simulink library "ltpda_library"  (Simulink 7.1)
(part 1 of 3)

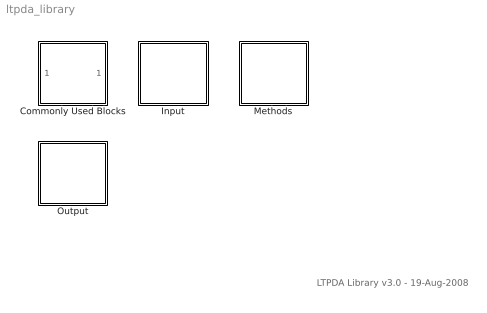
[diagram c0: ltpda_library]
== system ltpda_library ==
  note: LTPDA Library v3.0 - 19-Aug-2008
  Commonly Used Blocks : Subsystem
  Input : Subsystem
  Methods : Subsystem  Tag=subsystem  AncestorBlock=libraryBase/SubSystName
  Output : Subsystem

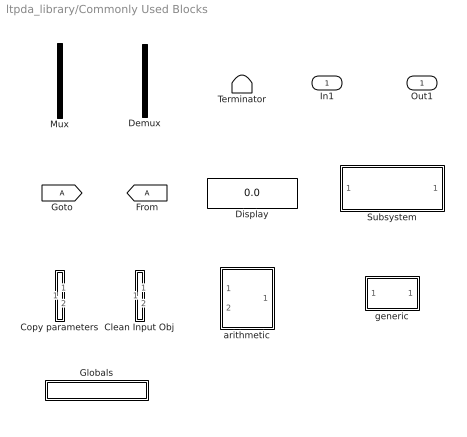
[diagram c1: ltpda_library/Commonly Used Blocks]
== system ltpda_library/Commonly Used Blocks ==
  In1 : Inport  OutDataType=sfix(16)  OutScaling=2^0
  Clean Input Obj : Subsystem
  Copy parameters : Subsystem
  Demux : Demux  Tag=demux  Outputs=2
  Display : Display
  Globals : Subsystem  Tag=globals
  Mux : Mux  Tag=mux  Inputs=2
  Subsystem : Subsystem
  Terminator : Terminator
  arithmetic : Subsystem  Tag=arithmetic
  generic : Subsystem  Tag=function
  Out1 : Outport  OutDataType=sfix(16)  OutScaling=2^0

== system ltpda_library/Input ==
  Object from list : Subsystem  Tag=input

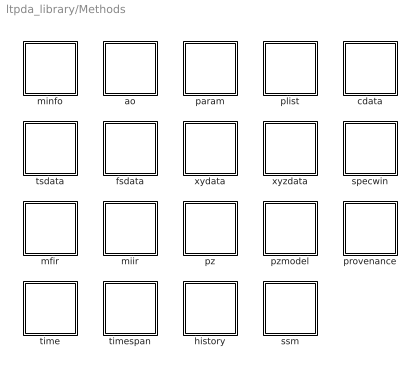
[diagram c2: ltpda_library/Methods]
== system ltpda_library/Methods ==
  ao : Subsystem  Tag=subsystem  AncestorBlock=libraryBase/SubSystName
  cdata : Subsystem  Tag=subsystem  AncestorBlock=libraryBase/SubSystName
  fsdata : Subsystem  Tag=subsystem  AncestorBlock=libraryBase/SubSystName
  history : Subsystem  Tag=subsystem  AncestorBlock=libraryBase/SubSystName
  mfir : Subsystem  Tag=subsystem  AncestorBlock=libraryBase/SubSystName
  miir : Subsystem  Tag=subsystem  AncestorBlock=libraryBase/SubSystName
  minfo : Subsystem  Tag=subsystem  AncestorBlock=libraryBase/SubSystName
  param : Subsystem  Tag=subsystem  AncestorBlock=libraryBase/SubSystName
  plist : Subsystem  Tag=subsystem  AncestorBlock=libraryBase/SubSystName
  provenance : Subsystem  Tag=subsystem  AncestorBlock=libraryBase/SubSystName
  pz : Subsystem  Tag=subsystem  AncestorBlock=libraryBase/SubSystName
  pzmodel : Subsystem  Tag=subsystem  AncestorBlock=libraryBase/SubSystName
  specwin : Subsystem  Tag=subsystem  AncestorBlock=libraryBase/SubSystName
  ssm : Subsystem  Tag=subsystem  AncestorBlock=libraryBase/SubSystName
  time : Subsystem  Tag=subsystem  AncestorBlock=libraryBase/SubSystName
  timespan : Subsystem  Tag=subsystem  AncestorBlock=libraryBase/SubSystName
  tsdata : Subsystem  Tag=subsystem  AncestorBlock=libraryBase/SubSystName
  xydata : Subsystem  Tag=subsystem  AncestorBlock=libraryBase/SubSystName
  xyzdata : Subsystem  Tag=subsystem  AncestorBlock=libraryBase/SubSystName

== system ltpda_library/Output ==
  Send to output : Subsystem
  iplot : Subsystem  Tag=method ao
  plot : Subsystem  Tag=method ao
  save : Subsystem  Tag=method ao

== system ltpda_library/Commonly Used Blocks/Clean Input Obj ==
  In1 : Inport  OutDataType=sfix(16)  OutScaling=2^0
  In2 : Inport  Port=2  OutDataType=sfix(16)  OutScaling=2^0
  cleaninput : M-S-Function  FunctionName=g_cleaninput
  Out1 : Outport  OutDataType=sfix(16)  OutScaling=2^0
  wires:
  In2/1 -> cleaninput/2
  In1/1 -> cleaninput/1
  cleaninput/1 -> Out1/1

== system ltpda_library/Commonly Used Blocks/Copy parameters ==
  In1 : Inport  OutDataType=sfix(16)  OutScaling=2^0
  In2 : Inport  Port=2  OutDataType=sfix(16)  OutScaling=2^0
  copyparam : M-S-Function  FunctionName=g_copyparams
  Out1 : Outport  OutDataType=sfix(16)  OutScaling=2^0
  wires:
  copyparam/1 -> Out1/1
  In1/1 -> copyparam/1
  In2/1 -> copyparam/2

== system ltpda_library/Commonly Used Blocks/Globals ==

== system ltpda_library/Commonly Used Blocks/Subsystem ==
  In1 : Inport  OutDataType=sfix(16)  OutScaling=2^0
  Out1 : Outport  OutDataType=sfix(16)  OutScaling=2^0

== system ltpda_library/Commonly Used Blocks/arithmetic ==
  alpha : Inport  Tag=1  OutDataType=sfix(16)  OutScaling=2^0
  beta : Inport  Tag=2  Port=2  OutDataType=sfix(16)  OutScaling=2^0
  Mux : Mux  Tag=mux  Inputs=2
  arithmetic_func : M-S-Function  Tag=arithmetic  FunctionName=ltpdasim
  Out1 : Outport  OutDataType=sfix(16)  OutScaling=2^0
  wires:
  arithmetic_func/1 -> Out1/1
  Mux/1 -> arithmetic_func/1
  alpha/1 -> Mux/1
  beta/1 -> Mux/2

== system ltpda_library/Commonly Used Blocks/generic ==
  In1 : Inport  OutDataType=sfix(16)  OutScaling=2^0
  generic : M-S-Function  Tag=generic  FunctionName=ltpdasim
  Out1 : Outport  OutDataType=sfix(16)  OutScaling=2^0
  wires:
  generic/1 -> Out1/1
  In1/1 -> generic/1

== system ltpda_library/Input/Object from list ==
  Input : Constant  Value=0  OutDataType=sfix(16)  OutScaling=2^0
  Input AO : Outport  OutDataType=sfix(16)  OutScaling=2^0
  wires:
  Input/1 -> Input AO/1

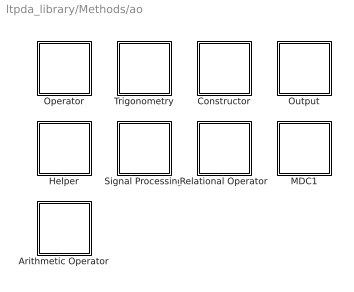
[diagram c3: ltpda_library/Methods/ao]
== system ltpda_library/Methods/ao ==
  Arithmetic Operator : Subsystem  Tag=subsystem  AncestorBlock=libraryBase/SubSystName
  Constructor : Subsystem  Tag=subsystem  AncestorBlock=libraryBase/SubSystName
  Helper : Subsystem  Tag=subsystem  AncestorBlock=libraryBase/SubSystName
  MDC1 : Subsystem  Tag=subsystem  AncestorBlock=libraryBase/SubSystName
  Operator : Subsystem  Tag=subsystem  AncestorBlock=libraryBase/SubSystName
  Output : Subsystem  Tag=subsystem  AncestorBlock=libraryBase/SubSystName
  Relational Operator : Subsystem  Tag=subsystem  AncestorBlock=libraryBase/SubSystName
  Signal Processing : Subsystem  Tag=subsystem  AncestorBlock=libraryBase/SubSystName
  Trigonometry : Subsystem  Tag=subsystem  AncestorBlock=libraryBase/SubSystName

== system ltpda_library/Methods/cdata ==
  Constructor : Subsystem  Tag=subsystem  AncestorBlock=libraryBase/SubSystName
  Helper : Subsystem  Tag=subsystem  AncestorBlock=libraryBase/SubSystName
  Output : Subsystem  Tag=subsystem  AncestorBlock=libraryBase/SubSystName
  Relational Operator : Subsystem  Tag=subsystem  AncestorBlock=libraryBase/SubSystName

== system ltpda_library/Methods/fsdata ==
  Constructor : Subsystem  Tag=subsystem  AncestorBlock=libraryBase/SubSystName
  Helper : Subsystem  Tag=subsystem  AncestorBlock=libraryBase/SubSystName
  Output : Subsystem  Tag=subsystem  AncestorBlock=libraryBase/SubSystName
  Relational Operator : Subsystem  Tag=subsystem  AncestorBlock=libraryBase/SubSystName

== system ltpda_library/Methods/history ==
  Constructor : Subsystem  Tag=subsystem  AncestorBlock=libraryBase/SubSystName
  Helper : Subsystem  Tag=subsystem  AncestorBlock=libraryBase/SubSystName
  Output : Subsystem  Tag=subsystem  AncestorBlock=libraryBase/SubSystName
  Relational Operator : Subsystem  Tag=subsystem  AncestorBlock=libraryBase/SubSystName

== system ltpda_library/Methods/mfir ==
  Constructor : Subsystem  Tag=subsystem  AncestorBlock=libraryBase/SubSystName
  Helper : Subsystem  Tag=subsystem  AncestorBlock=libraryBase/SubSystName
  Output : Subsystem  Tag=subsystem  AncestorBlock=libraryBase/SubSystName
  Relational Operator : Subsystem  Tag=subsystem  AncestorBlock=libraryBase/SubSystName
  Signal Processing : Subsystem  Tag=subsystem  AncestorBlock=libraryBase/SubSystName

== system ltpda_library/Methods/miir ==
  Constructor : Subsystem  Tag=subsystem  AncestorBlock=libraryBase/SubSystName
  Helper : Subsystem  Tag=subsystem  AncestorBlock=libraryBase/SubSystName
  Output : Subsystem  Tag=subsystem  AncestorBlock=libraryBase/SubSystName
  Relational Operator : Subsystem  Tag=subsystem  AncestorBlock=libraryBase/SubSystName
  Signal Processing : Subsystem  Tag=subsystem  AncestorBlock=libraryBase/SubSystName

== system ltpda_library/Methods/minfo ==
  Constructor : Subsystem  Tag=subsystem  AncestorBlock=libraryBase/SubSystName
  Helper : Subsystem  Tag=subsystem  AncestorBlock=libraryBase/SubSystName
  Output : Subsystem  Tag=subsystem  AncestorBlock=libraryBase/SubSystName
  Relational Operator : Subsystem  Tag=subsystem  AncestorBlock=libraryBase/SubSystName

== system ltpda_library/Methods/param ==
  Constructor : Subsystem  Tag=subsystem  AncestorBlock=libraryBase/SubSystName
  Helper : Subsystem  Tag=subsystem  AncestorBlock=libraryBase/SubSystName
  Output : Subsystem  Tag=subsystem  AncestorBlock=libraryBase/SubSystName
  Relational Operator : Subsystem  Tag=subsystem  AncestorBlock=libraryBase/SubSystName

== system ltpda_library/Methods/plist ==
  Constructor : Subsystem  Tag=subsystem  AncestorBlock=libraryBase/SubSystName
  Helper : Subsystem  Tag=subsystem  AncestorBlock=libraryBase/SubSystName
  Output : Subsystem  Tag=subsystem  AncestorBlock=libraryBase/SubSystName
  Relational Operator : Subsystem  Tag=subsystem  AncestorBlock=libraryBase/SubSystName
  Signal Processing : Subsystem  Tag=subsystem  AncestorBlock=libraryBase/SubSystName

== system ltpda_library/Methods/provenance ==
  Constructor : Subsystem  Tag=subsystem  AncestorBlock=libraryBase/SubSystName
  Helper : Subsystem  Tag=subsystem  AncestorBlock=libraryBase/SubSystName
  Output : Subsystem  Tag=subsystem  AncestorBlock=libraryBase/SubSystName
  Relational Operator : Subsystem  Tag=subsystem  AncestorBlock=libraryBase/SubSystName

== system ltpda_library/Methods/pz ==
  Constructor : Subsystem  Tag=subsystem  AncestorBlock=libraryBase/SubSystName
  Helper : Subsystem  Tag=subsystem  AncestorBlock=libraryBase/SubSystName
  Output : Subsystem  Tag=subsystem  AncestorBlock=libraryBase/SubSystName
  Relational Operator : Subsystem  Tag=subsystem  AncestorBlock=libraryBase/SubSystName
  Signal Processing : Subsystem  Tag=subsystem  AncestorBlock=libraryBase/SubSystName

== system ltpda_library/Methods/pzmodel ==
  Constructor : Subsystem  Tag=subsystem  AncestorBlock=libraryBase/SubSystName
  Helper : Subsystem  Tag=subsystem  AncestorBlock=libraryBase/SubSystName
  Operator : Subsystem  Tag=subsystem  AncestorBlock=libraryBase/SubSystName
  Output : Subsystem  Tag=subsystem  AncestorBlock=libraryBase/SubSystName
  Relational Operator : Subsystem  Tag=subsystem  AncestorBlock=libraryBase/SubSystName
  Signal Processing : Subsystem  Tag=subsystem  AncestorBlock=libraryBase/SubSystName

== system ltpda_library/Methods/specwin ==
  Constructor : Subsystem  Tag=subsystem  AncestorBlock=libraryBase/SubSystName
  Helper : Subsystem  Tag=subsystem  AncestorBlock=libraryBase/SubSystName
  Output : Subsystem  Tag=subsystem  AncestorBlock=libraryBase/SubSystName
  Relational Operator : Subsystem  Tag=subsystem  AncestorBlock=libraryBase/SubSystName

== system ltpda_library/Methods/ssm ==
  Constructor : Subsystem  Tag=subsystem  AncestorBlock=libraryBase/SubSystName
  Helper : Subsystem  Tag=subsystem  AncestorBlock=libraryBase/SubSystName
  Output : Subsystem  Tag=subsystem  AncestorBlock=libraryBase/SubSystName
  Relational Operator : Subsystem  Tag=subsystem  AncestorBlock=libraryBase/SubSystName
  STATESPACE : Subsystem  Tag=subsystem  AncestorBlock=libraryBase/SubSystName

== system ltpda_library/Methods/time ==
  Arithmetic Operator : Subsystem  Tag=subsystem  AncestorBlock=libraryBase/SubSystName
  Constructor : Subsystem  Tag=subsystem  AncestorBlock=libraryBase/SubSystName
  Helper : Subsystem  Tag=subsystem  AncestorBlock=libraryBase/SubSystName
  Output : Subsystem  Tag=subsystem  AncestorBlock=libraryBase/SubSystName
  Relational Operator : Subsystem  Tag=subsystem  AncestorBlock=libraryBase/SubSystName

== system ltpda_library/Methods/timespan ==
  Constructor : Subsystem  Tag=subsystem  AncestorBlock=libraryBase/SubSystName
  Helper : Subsystem  Tag=subsystem  AncestorBlock=libraryBase/SubSystName
  Output : Subsystem  Tag=subsystem  AncestorBlock=libraryBase/SubSystName
  Relational Operator : Subsystem  Tag=subsystem  AncestorBlock=libraryBase/SubSystName

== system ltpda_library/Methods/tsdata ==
  Constructor : Subsystem  Tag=subsystem  AncestorBlock=libraryBase/SubSystName
  Helper : Subsystem  Tag=subsystem  AncestorBlock=libraryBase/SubSystName
  Output : Subsystem  Tag=subsystem  AncestorBlock=libraryBase/SubSystName
  Relational Operator : Subsystem  Tag=subsystem  AncestorBlock=libraryBase/SubSystName

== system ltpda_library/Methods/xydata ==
  Constructor : Subsystem  Tag=subsystem  AncestorBlock=libraryBase/SubSystName
  Helper : Subsystem  Tag=subsystem  AncestorBlock=libraryBase/SubSystName
  Output : Subsystem  Tag=subsystem  AncestorBlock=libraryBase/SubSystName
  Relational Operator : Subsystem  Tag=subsystem  AncestorBlock=libraryBase/SubSystName

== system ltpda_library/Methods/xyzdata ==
  Constructor : Subsystem  Tag=subsystem  AncestorBlock=libraryBase/SubSystName
  Helper : Subsystem  Tag=subsystem  AncestorBlock=libraryBase/SubSystName
  Output : Subsystem  Tag=subsystem  AncestorBlock=libraryBase/SubSystName
  Relational Operator : Subsystem  Tag=subsystem  AncestorBlock=libraryBase/SubSystName

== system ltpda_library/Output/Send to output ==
  In1 : Inport  OutDataType=sfix(16)  OutScaling=2^0
  save result : M-S-Function  FunctionName=g_saveresult
  Out1 : Outport  OutDataType=sfix(16)  OutScaling=2^0
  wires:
  In1/1 -> save result/1
  save result/1 -> Out1/1

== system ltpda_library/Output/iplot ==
  In1 : Inport  OutDataType=sfix(16)  OutScaling=2^0
  Terminator : Terminator
  iplot : M-S-Function  Tag=iplot  FunctionName=ltpdasim
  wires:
  In1/1 -> iplot/1
  iplot/1 -> Terminator/1

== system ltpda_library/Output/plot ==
  In1 : Inport  OutDataType=sfix(16)  OutScaling=2^0
  Terminator : Terminator
  plot : M-S-Function  Tag=plot  FunctionName=ltpdasim
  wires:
  In1/1 -> plot/1
  plot/1 -> Terminator/1

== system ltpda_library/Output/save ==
  In1 : Inport  OutDataType=sfix(16)  OutScaling=2^0
  Terminator : Terminator
  save : M-S-Function  Tag=save  FunctionName=ltpdasim
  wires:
  In1/1 -> save/1
  save/1 -> Terminator/1

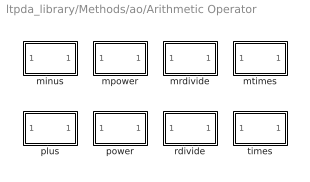
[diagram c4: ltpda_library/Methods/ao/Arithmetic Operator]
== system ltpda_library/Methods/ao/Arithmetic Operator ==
  minus : Subsystem  Tag=method ao  AncestorBlock=libraryBase/function
  mpower : Subsystem  Tag=method ao  AncestorBlock=libraryBase/function
  mrdivide : Subsystem  Tag=method ao  AncestorBlock=libraryBase/function
  mtimes : Subsystem  Tag=method ao  AncestorBlock=libraryBase/function
  plus : Subsystem  Tag=method ao  AncestorBlock=libraryBase/function
  power : Subsystem  Tag=method ao  AncestorBlock=libraryBase/function
  rdivide : Subsystem  Tag=method ao  AncestorBlock=libraryBase/function
  times : Subsystem  Tag=method ao  AncestorBlock=libraryBase/function

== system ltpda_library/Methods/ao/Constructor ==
  ao : Subsystem  Tag=method ao  AncestorBlock=libraryBase/constructor

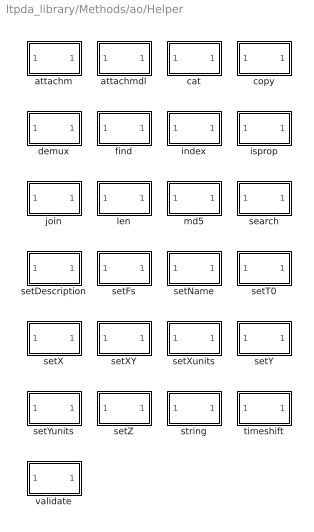
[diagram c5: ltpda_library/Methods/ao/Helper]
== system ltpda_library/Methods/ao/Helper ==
  attachm : Subsystem  Tag=method ao  AncestorBlock=libraryBase/function
  attachmdl : Subsystem  Tag=method ao  AncestorBlock=libraryBase/function
  cat : Subsystem  Tag=method ao  AncestorBlock=libraryBase/function
  copy : Subsystem  Tag=method ao  AncestorBlock=libraryBase/function
  demux : Subsystem  Tag=method ao  AncestorBlock=libraryBase/function
  find : Subsystem  Tag=method ao  AncestorBlock=libraryBase/function
  index : Subsystem  Tag=method ao  AncestorBlock=libraryBase/function
  isprop : Subsystem  Tag=method ao  AncestorBlock=libraryBase/function
  join : Subsystem  Tag=method ao  AncestorBlock=libraryBase/function
  len : Subsystem  Tag=method ao  AncestorBlock=libraryBase/function
  md5 : Subsystem  Tag=method ao  AncestorBlock=libraryBase/function
  search : Subsystem  Tag=method ao  AncestorBlock=libraryBase/function
  setDescription : Subsystem  Tag=method ao  AncestorBlock=libraryBase/function
  setFs : Subsystem  Tag=method ao  AncestorBlock=libraryBase/function
  setName : Subsystem  Tag=method ao  AncestorBlock=libraryBase/function
  setT0 : Subsystem  Tag=method ao  AncestorBlock=libraryBase/function
  setX : Subsystem  Tag=method ao  AncestorBlock=libraryBase/function
  setXY : Subsystem  Tag=method ao  AncestorBlock=libraryBase/function
  setXunits : Subsystem  Tag=method ao  AncestorBlock=libraryBase/function
  setY : Subsystem  Tag=method ao  AncestorBlock=libraryBase/function
  setYunits : Subsystem  Tag=method ao  AncestorBlock=libraryBase/function
  setZ : Subsystem  Tag=method ao  AncestorBlock=libraryBase/function
  string : Subsystem  Tag=method ao  AncestorBlock=libraryBase/function
  timeshift : Subsystem  Tag=method ao  AncestorBlock=libraryBase/function
  validate : Subsystem  Tag=method ao  AncestorBlock=libraryBase/function

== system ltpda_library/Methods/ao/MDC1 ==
  mdc1_ifo2acc_fd : Subsystem  Tag=method ao  AncestorBlock=libraryBase/function
  mdc1_ifo2acc_inloop : Subsystem  Tag=method ao  AncestorBlock=libraryBase/function
  mdc1_ifo2control : Subsystem  Tag=method ao  AncestorBlock=libraryBase/function
  mdc1_x2acc : Subsystem  Tag=method ao  AncestorBlock=libraryBase/function

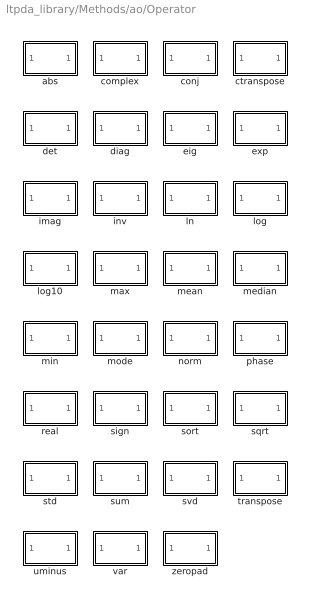
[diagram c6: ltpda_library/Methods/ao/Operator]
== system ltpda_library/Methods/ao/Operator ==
  abs : Subsystem  Tag=method ao  AncestorBlock=libraryBase/function
  complex : Subsystem  Tag=method ao  AncestorBlock=libraryBase/function
  conj : Subsystem  Tag=method ao  AncestorBlock=libraryBase/function
  ctranspose : Subsystem  Tag=method ao  AncestorBlock=libraryBase/function
  det : Subsystem  Tag=method ao  AncestorBlock=libraryBase/function
  diag : Subsystem  Tag=method ao  AncestorBlock=libraryBase/function
  eig : Subsystem  Tag=method ao  AncestorBlock=libraryBase/function
  exp : Subsystem  Tag=method ao  AncestorBlock=libraryBase/function
  imag : Subsystem  Tag=method ao  AncestorBlock=libraryBase/function
  inv : Subsystem  Tag=method ao  AncestorBlock=libraryBase/function
  ln : Subsystem  Tag=method ao  AncestorBlock=libraryBase/function
  log : Subsystem  Tag=method ao  AncestorBlock=libraryBase/function
  log10 : Subsystem  Tag=method ao  AncestorBlock=libraryBase/function
  max : Subsystem  Tag=method ao  AncestorBlock=libraryBase/function
  mean : Subsystem  Tag=method ao  AncestorBlock=libraryBase/function
  median : Subsystem  Tag=method ao  AncestorBlock=libraryBase/function
  min : Subsystem  Tag=method ao  AncestorBlock=libraryBase/function
  mode : Subsystem  Tag=method ao  AncestorBlock=libraryBase/function
  norm : Subsystem  Tag=method ao  AncestorBlock=libraryBase/function
  phase : Subsystem  Tag=method ao  AncestorBlock=libraryBase/function
  real : Subsystem  Tag=method ao  AncestorBlock=libraryBase/function
  sign : Subsystem  Tag=method ao  AncestorBlock=libraryBase/function
  sort : Subsystem  Tag=method ao  AncestorBlock=libraryBase/function
  sqrt : Subsystem  Tag=method ao  AncestorBlock=libraryBase/function
  std : Subsystem  Tag=method ao  AncestorBlock=libraryBase/function
  sum : Subsystem  Tag=method ao  AncestorBlock=libraryBase/function
  svd : Subsystem  Tag=method ao  AncestorBlock=libraryBase/function
  transpose : Subsystem  Tag=method ao  AncestorBlock=libraryBase/function
  uminus : Subsystem  Tag=method ao  AncestorBlock=libraryBase/function
  var : Subsystem  Tag=method ao  AncestorBlock=libraryBase/function
  zeropad : Subsystem  Tag=method ao  AncestorBlock=libraryBase/function

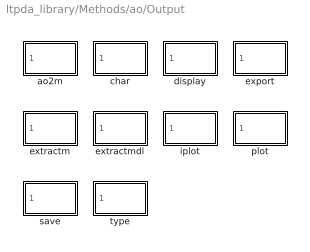
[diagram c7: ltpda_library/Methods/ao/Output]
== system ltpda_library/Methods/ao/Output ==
  ao2m : Subsystem  Tag=method ao  AncestorBlock=libraryBase/output
  char : Subsystem  Tag=method ao  AncestorBlock=libraryBase/output
  display : Subsystem  Tag=method ao  AncestorBlock=libraryBase/output
  export : Subsystem  Tag=method ao  AncestorBlock=libraryBase/output
  extractm : Subsystem  Tag=method ao  AncestorBlock=libraryBase/output
  extractmdl : Subsystem  Tag=method ao  AncestorBlock=libraryBase/output
  iplot : Subsystem  Tag=method ao  AncestorBlock=libraryBase/output
  plot : Subsystem  Tag=method ao  AncestorBlock=libraryBase/output
  save : Subsystem  Tag=method ao  AncestorBlock=libraryBase/output
  type : Subsystem  Tag=method ao  AncestorBlock=libraryBase/output

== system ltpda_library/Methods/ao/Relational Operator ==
  eq : Subsystem  Tag=method ao  AncestorBlock=libraryBase/function
  ge : Subsystem  Tag=method ao  AncestorBlock=libraryBase/function
  gt : Subsystem  Tag=method ao  AncestorBlock=libraryBase/function
  le : Subsystem  Tag=method ao  AncestorBlock=libraryBase/function
  lt : Subsystem  Tag=method ao  AncestorBlock=libraryBase/function
  ne : Subsystem  Tag=method ao  AncestorBlock=libraryBase/function

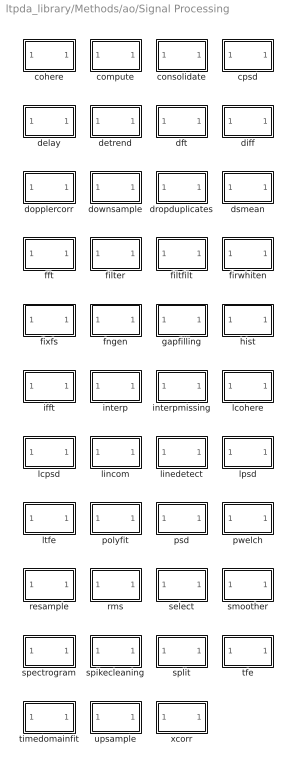
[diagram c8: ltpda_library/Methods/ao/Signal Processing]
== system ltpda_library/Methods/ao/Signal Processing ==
  cohere : Subsystem  Tag=method ao  AncestorBlock=libraryBase/function
  compute : Subsystem  Tag=method ao  AncestorBlock=libraryBase/function
  consolidate : Subsystem  Tag=method ao  AncestorBlock=libraryBase/function
  cpsd : Subsystem  Tag=method ao  AncestorBlock=libraryBase/function
  delay : Subsystem  Tag=method ao  AncestorBlock=libraryBase/function
  detrend : Subsystem  Tag=method ao  AncestorBlock=libraryBase/function
  dft : Subsystem  Tag=method ao  AncestorBlock=libraryBase/function
  diff : Subsystem  Tag=method ao  AncestorBlock=libraryBase/function
  dopplercorr : Subsystem  Tag=method ao  AncestorBlock=libraryBase/function
  downsample : Subsystem  Tag=method ao  AncestorBlock=libraryBase/function
  dropduplicates : Subsystem  Tag=method ao  AncestorBlock=libraryBase/function
  dsmean : Subsystem  Tag=method ao  AncestorBlock=libraryBase/function
  fft : Subsystem  Tag=method ao  AncestorBlock=libraryBase/function
  filter : Subsystem  Tag=method ao  AncestorBlock=libraryBase/function
  filtfilt : Subsystem  Tag=method ao  AncestorBlock=libraryBase/function
  firwhiten : Subsystem  Tag=method ao  AncestorBlock=libraryBase/function
  fixfs : Subsystem  Tag=method ao  AncestorBlock=libraryBase/function
  fngen : Subsystem  Tag=method ao  AncestorBlock=libraryBase/function
  gapfilling : Subsystem  Tag=method ao  AncestorBlock=libraryBase/function
  hist : Subsystem  Tag=method ao  AncestorBlock=libraryBase/function
  ifft : Subsystem  Tag=method ao  AncestorBlock=libraryBase/function
  interp : Subsystem  Tag=method ao  AncestorBlock=libraryBase/function
  interpmissing : Subsystem  Tag=method ao  AncestorBlock=libraryBase/function
  lcohere : Subsystem  Tag=method ao  AncestorBlock=libraryBase/function
  lcpsd : Subsystem  Tag=method ao  AncestorBlock=libraryBase/function
  lincom : Subsystem  Tag=method ao  AncestorBlock=libraryBase/function
  linedetect : Subsystem  Tag=method ao  AncestorBlock=libraryBase/function
  lpsd : Subsystem  Tag=method ao  AncestorBlock=libraryBase/function
  ltfe : Subsystem  Tag=method ao  AncestorBlock=libraryBase/function
  polyfit : Subsystem  Tag=method ao  AncestorBlock=libraryBase/function
  psd : Subsystem  Tag=method ao  AncestorBlock=libraryBase/function
  pwelch : Subsystem  Tag=method ao  AncestorBlock=libraryBase/function
  resample : Subsystem  Tag=method ao  AncestorBlock=libraryBase/function
  rms : Subsystem  Tag=method ao  AncestorBlock=libraryBase/function
  select : Subsystem  Tag=method ao  AncestorBlock=libraryBase/function
  smoother : Subsystem  Tag=method ao  AncestorBlock=libraryBase/function
  spectrogram : Subsystem  Tag=method ao  AncestorBlock=libraryBase/function
  spikecleaning : Subsystem  Tag=method ao  AncestorBlock=libraryBase/function
  split : Subsystem  Tag=method ao  AncestorBlock=libraryBase/function
  tfe : Subsystem  Tag=method ao  AncestorBlock=libraryBase/function
  timedomainfit : Subsystem  Tag=method ao  AncestorBlock=libraryBase/function
  upsample : Subsystem  Tag=method ao  AncestorBlock=libraryBase/function
  xcorr : Subsystem  Tag=method ao  AncestorBlock=libraryBase/function

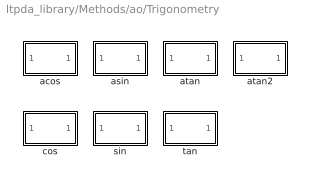
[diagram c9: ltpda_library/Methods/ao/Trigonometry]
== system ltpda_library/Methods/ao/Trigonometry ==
  acos : Subsystem  Tag=method ao  AncestorBlock=libraryBase/function
  asin : Subsystem  Tag=method ao  AncestorBlock=libraryBase/function
  atan : Subsystem  Tag=method ao  AncestorBlock=libraryBase/function
  atan2 : Subsystem  Tag=method ao  AncestorBlock=libraryBase/function
  cos : Subsystem  Tag=method ao  AncestorBlock=libraryBase/function
  sin : Subsystem  Tag=method ao  AncestorBlock=libraryBase/function
  tan : Subsystem  Tag=method ao  AncestorBlock=libraryBase/function

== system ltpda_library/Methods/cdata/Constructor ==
  cdata : Subsystem  Tag=method cdata  AncestorBlock=libraryBase/constructor

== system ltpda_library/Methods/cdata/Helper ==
  isprop : Subsystem  Tag=method cdata  AncestorBlock=libraryBase/function

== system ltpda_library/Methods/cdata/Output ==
  display : Subsystem  Tag=method cdata  AncestorBlock=libraryBase/output

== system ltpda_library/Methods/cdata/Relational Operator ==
  eq : Subsystem  Tag=method cdata  AncestorBlock=libraryBase/function
  ne : Subsystem  Tag=method cdata  AncestorBlock=libraryBase/function

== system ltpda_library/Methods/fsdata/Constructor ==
  fsdata : Subsystem  Tag=method fsdata  AncestorBlock=libraryBase/constructor

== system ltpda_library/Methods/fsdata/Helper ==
  isprop : Subsystem  Tag=method fsdata  AncestorBlock=libraryBase/function

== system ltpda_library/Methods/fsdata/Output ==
  char : Subsystem  Tag=method fsdata  AncestorBlock=libraryBase/output
  display : Subsystem  Tag=method fsdata  AncestorBlock=libraryBase/output

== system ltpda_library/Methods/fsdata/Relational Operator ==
  eq : Subsystem  Tag=method fsdata  AncestorBlock=libraryBase/function
  ne : Subsystem  Tag=method fsdata  AncestorBlock=libraryBase/function

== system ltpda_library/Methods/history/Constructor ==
  history : Subsystem  Tag=method history  AncestorBlock=libraryBase/constructor

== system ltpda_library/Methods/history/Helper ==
  isprop : Subsystem  Tag=method history  AncestorBlock=libraryBase/function

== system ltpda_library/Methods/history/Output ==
  char : Subsystem  Tag=method history  AncestorBlock=libraryBase/output
  display : Subsystem  Tag=method history  AncestorBlock=libraryBase/output
  hist2dot : Subsystem  Tag=method history  AncestorBlock=libraryBase/output
  hist2m : Subsystem  Tag=method history  AncestorBlock=libraryBase/output
  plot : Subsystem  Tag=method history  AncestorBlock=libraryBase/output
  string : Subsystem  Tag=method history  AncestorBlock=libraryBase/output

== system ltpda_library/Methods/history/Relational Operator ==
  eq : Subsystem  Tag=method history  AncestorBlock=libraryBase/function
  ne : Subsystem  Tag=method history  AncestorBlock=libraryBase/function

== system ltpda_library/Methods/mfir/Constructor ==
  mfir : Subsystem  Tag=method mfir  AncestorBlock=libraryBase/constructor

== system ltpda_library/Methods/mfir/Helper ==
  isprop : Subsystem  Tag=method mfir  AncestorBlock=libraryBase/function
  redesign : Subsystem  Tag=method mfir  AncestorBlock=libraryBase/function
  setName : Subsystem  Tag=method mfir  AncestorBlock=libraryBase/function

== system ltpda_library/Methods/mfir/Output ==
  char : Subsystem  Tag=method mfir  AncestorBlock=libraryBase/output
  display : Subsystem  Tag=method mfir  AncestorBlock=libraryBase/output
  save : Subsystem  Tag=method mfir  AncestorBlock=libraryBase/output
  string : Subsystem  Tag=method mfir  AncestorBlock=libraryBase/output

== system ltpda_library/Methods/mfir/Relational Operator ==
  eq : Subsystem  Tag=method mfir  AncestorBlock=libraryBase/function
  ne : Subsystem  Tag=method mfir  AncestorBlock=libraryBase/function

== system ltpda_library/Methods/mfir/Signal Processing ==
  resp : Subsystem  Tag=method mfir  AncestorBlock=libraryBase/function

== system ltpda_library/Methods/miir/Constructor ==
  miir : Subsystem  Tag=method miir  AncestorBlock=libraryBase/constructor

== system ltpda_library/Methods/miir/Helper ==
  isprop : Subsystem  Tag=method miir  AncestorBlock=libraryBase/function
  redesign : Subsystem  Tag=method miir  AncestorBlock=libraryBase/function
  setName : Subsystem  Tag=method miir  AncestorBlock=libraryBase/function

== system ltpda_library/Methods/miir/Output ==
  char : Subsystem  Tag=method miir  AncestorBlock=libraryBase/output
  display : Subsystem  Tag=method miir  AncestorBlock=libraryBase/output
  save : Subsystem  Tag=method miir  AncestorBlock=libraryBase/output
  string : Subsystem  Tag=method miir  AncestorBlock=libraryBase/output

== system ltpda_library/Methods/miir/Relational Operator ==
  eq : Subsystem  Tag=method miir  AncestorBlock=libraryBase/function
  ne : Subsystem  Tag=method miir  AncestorBlock=libraryBase/function

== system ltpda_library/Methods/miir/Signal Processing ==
  resp : Subsystem  Tag=method miir  AncestorBlock=libraryBase/function

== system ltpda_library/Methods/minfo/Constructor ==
  minfo : Subsystem  Tag=method minfo  AncestorBlock=libraryBase/constructor

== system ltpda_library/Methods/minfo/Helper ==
  isprop : Subsystem  Tag=method minfo  AncestorBlock=libraryBase/function

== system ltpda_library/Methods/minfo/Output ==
  char : Subsystem  Tag=method minfo  AncestorBlock=libraryBase/output
  display : Subsystem  Tag=method minfo  AncestorBlock=libraryBase/output

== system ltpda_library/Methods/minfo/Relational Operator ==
  eq : Subsystem  Tag=method minfo  AncestorBlock=libraryBase/function
  ne : Subsystem  Tag=method minfo  AncestorBlock=libraryBase/function

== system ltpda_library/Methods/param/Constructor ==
  param : Subsystem  Tag=method param  AncestorBlock=libraryBase/constructor

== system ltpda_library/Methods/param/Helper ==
  isprop : Subsystem  Tag=method param  AncestorBlock=libraryBase/function
  mux : Subsystem  Tag=method param  AncestorBlock=libraryBase/function

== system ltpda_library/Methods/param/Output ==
  char : Subsystem  Tag=method param  AncestorBlock=libraryBase/output
  display : Subsystem  Tag=method param  AncestorBlock=libraryBase/output
  display2 : Subsystem  Tag=method param  AncestorBlock=libraryBase/output
  string : Subsystem  Tag=method param  AncestorBlock=libraryBase/output

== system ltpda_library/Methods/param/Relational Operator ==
  eq : Subsystem  Tag=method param  AncestorBlock=libraryBase/function
  ne : Subsystem  Tag=method param  AncestorBlock=libraryBase/function

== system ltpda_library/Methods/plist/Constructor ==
  plist : Subsystem  Tag=method plist  AncestorBlock=libraryBase/constructor

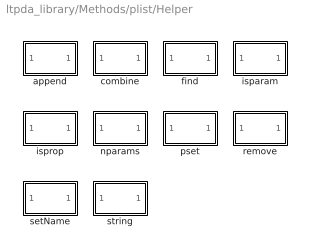
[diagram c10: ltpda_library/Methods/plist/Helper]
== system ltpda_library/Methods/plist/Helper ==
  append : Subsystem  Tag=method plist  AncestorBlock=libraryBase/function
  combine : Subsystem  Tag=method plist  AncestorBlock=libraryBase/function
  find : Subsystem  Tag=method plist  AncestorBlock=libraryBase/function
  isparam : Subsystem  Tag=method plist  AncestorBlock=libraryBase/function
  isprop : Subsystem  Tag=method plist  AncestorBlock=libraryBase/function
  nparams : Subsystem  Tag=method plist  AncestorBlock=libraryBase/function
  pset : Subsystem  Tag=method plist  AncestorBlock=libraryBase/function
  remove : Subsystem  Tag=method plist  AncestorBlock=libraryBase/function
  setName : Subsystem  Tag=method plist  AncestorBlock=libraryBase/function
  string : Subsystem  Tag=method plist  AncestorBlock=libraryBase/function

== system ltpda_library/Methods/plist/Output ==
  char : Subsystem  Tag=method plist  AncestorBlock=libraryBase/output
  display : Subsystem  Tag=method plist  AncestorBlock=libraryBase/output
  save : Subsystem  Tag=method plist  AncestorBlock=libraryBase/output

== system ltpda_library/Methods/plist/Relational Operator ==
  eq : Subsystem  Tag=method plist  AncestorBlock=libraryBase/function
  ne : Subsystem  Tag=method plist  AncestorBlock=libraryBase/function

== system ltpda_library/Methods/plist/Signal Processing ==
  resp : Subsystem  Tag=method plist  AncestorBlock=libraryBase/function

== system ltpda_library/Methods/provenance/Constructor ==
  provenance : Subsystem  Tag=method provenance  AncestorBlock=libraryBase/constructor

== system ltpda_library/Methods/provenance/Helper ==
  isprop : Subsystem  Tag=method provenance  AncestorBlock=libraryBase/function

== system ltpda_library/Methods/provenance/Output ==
  char : Subsystem  Tag=method provenance  AncestorBlock=libraryBase/output
  display : Subsystem  Tag=method provenance  AncestorBlock=libraryBase/output
  string : Subsystem  Tag=method provenance  AncestorBlock=libraryBase/output

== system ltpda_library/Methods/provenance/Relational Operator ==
  eq : Subsystem  Tag=method provenance  AncestorBlock=libraryBase/function
  ne : Subsystem  Tag=method provenance  AncestorBlock=libraryBase/function

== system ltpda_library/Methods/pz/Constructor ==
  pz : Subsystem  Tag=method pz  AncestorBlock=libraryBase/constructor

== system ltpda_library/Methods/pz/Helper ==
  isprop : Subsystem  Tag=method pz  AncestorBlock=libraryBase/function

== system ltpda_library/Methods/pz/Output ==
  char : Subsystem  Tag=method pz  AncestorBlock=libraryBase/output
  display : Subsystem  Tag=method pz  AncestorBlock=libraryBase/output
  string : Subsystem  Tag=method pz  AncestorBlock=libraryBase/output

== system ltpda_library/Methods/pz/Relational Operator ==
  eq : Subsystem  Tag=method pz  AncestorBlock=libraryBase/function
  ne : Subsystem  Tag=method pz  AncestorBlock=libraryBase/function

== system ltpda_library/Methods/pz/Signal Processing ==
  resp : Subsystem  Tag=method pz  AncestorBlock=libraryBase/function

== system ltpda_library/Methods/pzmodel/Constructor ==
  pzmodel : Subsystem  Tag=method pzmodel  AncestorBlock=libraryBase/constructor

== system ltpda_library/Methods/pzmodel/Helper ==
  isprop : Subsystem  Tag=method pzmodel  AncestorBlock=libraryBase/function
  setName : Subsystem  Tag=method pzmodel  AncestorBlock=libraryBase/function
  string : Subsystem  Tag=method pzmodel  AncestorBlock=libraryBase/function

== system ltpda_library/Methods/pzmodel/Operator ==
  tomfir : Subsystem  Tag=method pzmodel  AncestorBlock=libraryBase/function
  tomiir : Subsystem  Tag=method pzmodel  AncestorBlock=libraryBase/function

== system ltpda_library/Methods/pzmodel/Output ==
  char : Subsystem  Tag=method pzmodel  AncestorBlock=libraryBase/output
  display : Subsystem  Tag=method pzmodel  AncestorBlock=libraryBase/output
  save : Subsystem  Tag=method pzmodel  AncestorBlock=libraryBase/output

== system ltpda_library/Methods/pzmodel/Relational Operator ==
  eq : Subsystem  Tag=method pzmodel  AncestorBlock=libraryBase/function
  ne : Subsystem  Tag=method pzmodel  AncestorBlock=libraryBase/function

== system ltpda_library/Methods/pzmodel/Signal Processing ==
  fngen : Subsystem  Tag=method pzmodel  AncestorBlock=libraryBase/function
  resp : Subsystem  Tag=method pzmodel  AncestorBlock=libraryBase/function

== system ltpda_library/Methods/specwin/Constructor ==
  specwin : Subsystem  Tag=method specwin  AncestorBlock=libraryBase/constructor

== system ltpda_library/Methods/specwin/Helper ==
  isprop : Subsystem  Tag=method specwin  AncestorBlock=libraryBase/function

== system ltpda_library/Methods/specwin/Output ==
  char : Subsystem  Tag=method specwin  AncestorBlock=libraryBase/output
  display : Subsystem  Tag=method specwin  AncestorBlock=libraryBase/output
  plot : Subsystem  Tag=method specwin  AncestorBlock=libraryBase/output
  string : Subsystem  Tag=method specwin  AncestorBlock=libraryBase/output

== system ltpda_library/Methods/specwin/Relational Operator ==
  eq : Subsystem  Tag=method specwin  AncestorBlock=libraryBase/function
  ne : Subsystem  Tag=method specwin  AncestorBlock=libraryBase/function

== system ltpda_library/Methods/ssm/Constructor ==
  ssm : Subsystem  Tag=method ssm  AncestorBlock=libraryBase/constructor

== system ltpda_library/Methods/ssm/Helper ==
  isprop : Subsystem  Tag=method ssm  AncestorBlock=libraryBase/function
  setName : Subsystem  Tag=method ssm  AncestorBlock=libraryBase/function

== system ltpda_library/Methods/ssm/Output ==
  char : Subsystem  Tag=method ssm  AncestorBlock=libraryBase/output
  display : Subsystem  Tag=method ssm  AncestorBlock=libraryBase/output
  isstable : Subsystem  Tag=method ssm  AncestorBlock=libraryBase/output
  save : Subsystem  Tag=method ssm  AncestorBlock=libraryBase/output
  string : Subsystem  Tag=method ssm  AncestorBlock=libraryBase/output

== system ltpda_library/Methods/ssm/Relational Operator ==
  eq : Subsystem  Tag=method ssm  AncestorBlock=libraryBase/function
  ne : Subsystem  Tag=method ssm  AncestorBlock=libraryBase/function

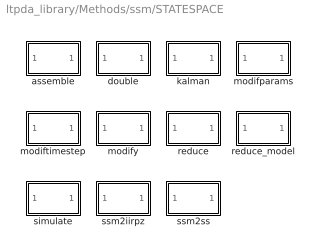
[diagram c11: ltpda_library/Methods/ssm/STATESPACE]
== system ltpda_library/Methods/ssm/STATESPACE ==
  assemble : Subsystem  Tag=method ssm  AncestorBlock=libraryBase/function
  double : Subsystem  Tag=method ssm  AncestorBlock=libraryBase/function
  kalman : Subsystem  Tag=method ssm  AncestorBlock=libraryBase/function
  modifparams : Subsystem  Tag=method ssm  AncestorBlock=libraryBase/function
  modiftimestep : Subsystem  Tag=method ssm  AncestorBlock=libraryBase/function
  modify : Subsystem  Tag=method ssm  AncestorBlock=libraryBase/function
  reduce : Subsystem  Tag=method ssm  AncestorBlock=libraryBase/function
  reduce_model : Subsystem  Tag=method ssm  AncestorBlock=libraryBase/function
  simulate : Subsystem  Tag=method ssm  AncestorBlock=libraryBase/function
  ssm2iirpz : Subsystem  Tag=method ssm  AncestorBlock=libraryBase/function
  ssm2ss : Subsystem  Tag=method ssm  AncestorBlock=libraryBase/function

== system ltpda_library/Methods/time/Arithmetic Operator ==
  minus : Subsystem  Tag=method time  AncestorBlock=libraryBase/function
  plus : Subsystem  Tag=method time  AncestorBlock=libraryBase/function

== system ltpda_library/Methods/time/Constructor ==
  time : Subsystem  Tag=method time  AncestorBlock=libraryBase/constructor

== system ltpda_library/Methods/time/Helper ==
  getTimezones : Subsystem  Tag=method time  AncestorBlock=libraryBase/function
  isprop : Subsystem  Tag=method time  AncestorBlock=libraryBase/function
  string : Subsystem  Tag=method time  AncestorBlock=libraryBase/function

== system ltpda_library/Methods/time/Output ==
  char : Subsystem  Tag=method time  AncestorBlock=libraryBase/output
  display : Subsystem  Tag=method time  AncestorBlock=libraryBase/output
  format : Subsystem  Tag=method time  AncestorBlock=libraryBase/output

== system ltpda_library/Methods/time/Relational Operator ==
  eq : Subsystem  Tag=method time  AncestorBlock=libraryBase/function
  ne : Subsystem  Tag=method time  AncestorBlock=libraryBase/function

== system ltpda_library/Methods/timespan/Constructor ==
  timespan : Subsystem  Tag=method timespan  AncestorBlock=libraryBase/constructor

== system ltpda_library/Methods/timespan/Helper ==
  isprop : Subsystem  Tag=method timespan  AncestorBlock=libraryBase/function
  setEndT : Subsystem  Tag=method timespan  AncestorBlock=libraryBase/function
  setName : Subsystem  Tag=method timespan  AncestorBlock=libraryBase/function
  setStartT : Subsystem  Tag=method timespan  AncestorBlock=libraryBase/function
  setTimeformat : Subsystem  Tag=method timespan  AncestorBlock=libraryBase/function
  setTimezone : Subsystem  Tag=method timespan  AncestorBlock=libraryBase/function

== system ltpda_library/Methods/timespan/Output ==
  char : Subsystem  Tag=method timespan  AncestorBlock=libraryBase/output
  display : Subsystem  Tag=method timespan  AncestorBlock=libraryBase/output
  save : Subsystem  Tag=method timespan  AncestorBlock=libraryBase/output
  string : Subsystem  Tag=method timespan  AncestorBlock=libraryBase/output

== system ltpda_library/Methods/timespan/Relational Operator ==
  eq : Subsystem  Tag=method timespan  AncestorBlock=libraryBase/function
  ne : Subsystem  Tag=method timespan  AncestorBlock=libraryBase/function

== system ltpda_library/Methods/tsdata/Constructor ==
  tsdata : Subsystem  Tag=method tsdata  AncestorBlock=libraryBase/constructor

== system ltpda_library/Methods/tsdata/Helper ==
  isprop : Subsystem  Tag=method tsdata  AncestorBlock=libraryBase/function

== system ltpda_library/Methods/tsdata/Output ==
  char : Subsystem  Tag=method tsdata  AncestorBlock=libraryBase/output
  display : Subsystem  Tag=method tsdata  AncestorBlock=libraryBase/output

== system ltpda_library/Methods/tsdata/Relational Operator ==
  eq : Subsystem  Tag=method tsdata  AncestorBlock=libraryBase/function
  ne : Subsystem  Tag=method tsdata  AncestorBlock=libraryBase/function

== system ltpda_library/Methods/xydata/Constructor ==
  xydata : Subsystem  Tag=method xydata  AncestorBlock=libraryBase/constructor

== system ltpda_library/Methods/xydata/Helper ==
  isprop : Subsystem  Tag=method xydata  AncestorBlock=libraryBase/function

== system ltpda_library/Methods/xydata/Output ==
  char : Subsystem  Tag=method xydata  AncestorBlock=libraryBase/output
  display : Subsystem  Tag=method xydata  AncestorBlock=libraryBase/output

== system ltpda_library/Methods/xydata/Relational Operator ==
  eq : Subsystem  Tag=method xydata  AncestorBlock=libraryBase/function
  ne : Subsystem  Tag=method xydata  AncestorBlock=libraryBase/function

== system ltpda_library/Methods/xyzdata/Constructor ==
  xyzdata : Subsystem  Tag=method xyzdata  AncestorBlock=libraryBase/constructor

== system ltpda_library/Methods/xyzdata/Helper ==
  isprop : Subsystem  Tag=method xyzdata  AncestorBlock=libraryBase/function

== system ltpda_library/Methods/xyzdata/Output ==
  char : Subsystem  Tag=method xyzdata  AncestorBlock=libraryBase/output
  display : Subsystem  Tag=method xyzdata  AncestorBlock=libraryBase/output

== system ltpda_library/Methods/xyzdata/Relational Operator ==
  eq : Subsystem  Tag=method xyzdata  AncestorBlock=libraryBase/function
  ne : Subsystem  Tag=method xyzdata  AncestorBlock=libraryBase/function

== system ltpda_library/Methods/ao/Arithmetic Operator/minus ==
  In1 : Inport  OutDataType=sfix(16)  OutScaling=2^0
  minus : M-S-Function  Tag=minus  FunctionName=ltpdasim
  Out1 : Outport  OutDataType=sfix(16)  OutScaling=2^0
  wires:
  In1/1 -> minus/1
  minus/1 -> Out1/1

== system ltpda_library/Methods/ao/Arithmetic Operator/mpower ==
  In1 : Inport  OutDataType=sfix(16)  OutScaling=2^0
  mpower : M-S-Function  Tag=mpower  FunctionName=ltpdasim
  Out1 : Outport  OutDataType=sfix(16)  OutScaling=2^0
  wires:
  In1/1 -> mpower/1
  mpower/1 -> Out1/1

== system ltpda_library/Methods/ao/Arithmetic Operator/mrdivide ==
  In1 : Inport  OutDataType=sfix(16)  OutScaling=2^0
  mrdivide : M-S-Function  Tag=mrdivide  FunctionName=ltpdasim
  Out1 : Outport  OutDataType=sfix(16)  OutScaling=2^0
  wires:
  In1/1 -> mrdivide/1
  mrdivide/1 -> Out1/1

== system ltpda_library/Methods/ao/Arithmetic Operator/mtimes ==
  In1 : Inport  OutDataType=sfix(16)  OutScaling=2^0
  mtimes : M-S-Function  Tag=mtimes  FunctionName=ltpdasim
  Out1 : Outport  OutDataType=sfix(16)  OutScaling=2^0
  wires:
  In1/1 -> mtimes/1
  mtimes/1 -> Out1/1

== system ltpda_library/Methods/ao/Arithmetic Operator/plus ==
  In1 : Inport  OutDataType=sfix(16)  OutScaling=2^0
  plus : M-S-Function  Tag=plus  FunctionName=ltpdasim
  Out1 : Outport  OutDataType=sfix(16)  OutScaling=2^0
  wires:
  In1/1 -> plus/1
  plus/1 -> Out1/1

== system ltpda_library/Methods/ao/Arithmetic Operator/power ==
  In1 : Inport  OutDataType=sfix(16)  OutScaling=2^0
  power : M-S-Function  Tag=power  FunctionName=ltpdasim
  Out1 : Outport  OutDataType=sfix(16)  OutScaling=2^0
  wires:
  In1/1 -> power/1
  power/1 -> Out1/1

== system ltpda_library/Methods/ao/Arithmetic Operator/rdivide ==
  In1 : Inport  OutDataType=sfix(16)  OutScaling=2^0
  rdivide : M-S-Function  Tag=rdivide  FunctionName=ltpdasim
  Out1 : Outport  OutDataType=sfix(16)  OutScaling=2^0
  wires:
  In1/1 -> rdivide/1
  rdivide/1 -> Out1/1

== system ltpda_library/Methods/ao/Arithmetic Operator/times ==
  In1 : Inport  OutDataType=sfix(16)  OutScaling=2^0
  times : M-S-Function  Tag=times  FunctionName=ltpdasim
  Out1 : Outport  OutDataType=sfix(16)  OutScaling=2^0
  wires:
  In1/1 -> times/1
  times/1 -> Out1/1

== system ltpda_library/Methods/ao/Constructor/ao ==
  Ground : Ground
  ao : M-S-Function  Tag=ao  FunctionName=ltpdasim
  Out1 : Outport  OutDataType=sfix(16)  OutScaling=2^0
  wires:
  Ground/1 -> ao/1
  ao/1 -> Out1/1

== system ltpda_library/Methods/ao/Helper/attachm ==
  In1 : Inport  OutDataType=sfix(16)  OutScaling=2^0
  attachm : M-S-Function  Tag=attachm  FunctionName=ltpdasim
  Out1 : Outport  OutDataType=sfix(16)  OutScaling=2^0
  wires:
  In1/1 -> attachm/1
  attachm/1 -> Out1/1

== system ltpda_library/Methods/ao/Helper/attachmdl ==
  In1 : Inport  OutDataType=sfix(16)  OutScaling=2^0
  attachmdl : M-S-Function  Tag=attachmdl  FunctionName=ltpdasim
  Out1 : Outport  OutDataType=sfix(16)  OutScaling=2^0
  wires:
  In1/1 -> attachmdl/1
  attachmdl/1 -> Out1/1

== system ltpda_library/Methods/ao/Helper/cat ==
  In1 : Inport  OutDataType=sfix(16)  OutScaling=2^0
  cat : M-S-Function  Tag=cat  FunctionName=ltpdasim
  Out1 : Outport  OutDataType=sfix(16)  OutScaling=2^0
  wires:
  In1/1 -> cat/1
  cat/1 -> Out1/1

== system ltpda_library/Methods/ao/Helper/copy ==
  In1 : Inport  OutDataType=sfix(16)  OutScaling=2^0
  copy : M-S-Function  Tag=copy  FunctionName=ltpdasim
  Out1 : Outport  OutDataType=sfix(16)  OutScaling=2^0
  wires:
  In1/1 -> copy/1
  copy/1 -> Out1/1

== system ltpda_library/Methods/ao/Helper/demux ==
  In1 : Inport  OutDataType=sfix(16)  OutScaling=2^0
  demux : M-S-Function  Tag=demux  FunctionName=ltpdasim
  Out1 : Outport  OutDataType=sfix(16)  OutScaling=2^0
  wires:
  In1/1 -> demux/1
  demux/1 -> Out1/1

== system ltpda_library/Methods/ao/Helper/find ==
  In1 : Inport  OutDataType=sfix(16)  OutScaling=2^0
  find : M-S-Function  Tag=find  FunctionName=ltpdasim
  Out1 : Outport  OutDataType=sfix(16)  OutScaling=2^0
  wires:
  In1/1 -> find/1
  find/1 -> Out1/1

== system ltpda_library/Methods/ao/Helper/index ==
  In1 : Inport  OutDataType=sfix(16)  OutScaling=2^0
  index : M-S-Function  Tag=index  FunctionName=ltpdasim
  Out1 : Outport  OutDataType=sfix(16)  OutScaling=2^0
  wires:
  In1/1 -> index/1
  index/1 -> Out1/1

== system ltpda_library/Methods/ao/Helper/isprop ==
  In1 : Inport  OutDataType=sfix(16)  OutScaling=2^0
  isprop : M-S-Function  Tag=isprop  FunctionName=ltpdasim
  Out1 : Outport  OutDataType=sfix(16)  OutScaling=2^0
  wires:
  In1/1 -> isprop/1
  isprop/1 -> Out1/1

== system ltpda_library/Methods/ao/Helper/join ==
  In1 : Inport  OutDataType=sfix(16)  OutScaling=2^0
  join : M-S-Function  Tag=join  FunctionName=ltpdasim
  Out1 : Outport  OutDataType=sfix(16)  OutScaling=2^0
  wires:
  In1/1 -> join/1
  join/1 -> Out1/1

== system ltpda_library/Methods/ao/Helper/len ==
  In1 : Inport  OutDataType=sfix(16)  OutScaling=2^0
  len : M-S-Function  Tag=len  FunctionName=ltpdasim
  Out1 : Outport  OutDataType=sfix(16)  OutScaling=2^0
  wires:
  In1/1 -> len/1
  len/1 -> Out1/1

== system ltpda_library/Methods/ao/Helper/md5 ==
  In1 : Inport  OutDataType=sfix(16)  OutScaling=2^0
  md5 : M-S-Function  Tag=md5  FunctionName=ltpdasim
  Out1 : Outport  OutDataType=sfix(16)  OutScaling=2^0
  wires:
  In1/1 -> md5/1
  md5/1 -> Out1/1

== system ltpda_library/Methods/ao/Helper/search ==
  In1 : Inport  OutDataType=sfix(16)  OutScaling=2^0
  search : M-S-Function  Tag=search  FunctionName=ltpdasim
  Out1 : Outport  OutDataType=sfix(16)  OutScaling=2^0
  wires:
  In1/1 -> search/1
  search/1 -> Out1/1

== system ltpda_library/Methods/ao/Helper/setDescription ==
  In1 : Inport  OutDataType=sfix(16)  OutScaling=2^0
  setDescription : M-S-Function  Tag=setDescription  FunctionName=ltpdasim
  Out1 : Outport  OutDataType=sfix(16)  OutScaling=2^0
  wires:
  In1/1 -> setDescription/1
  setDescription/1 -> Out1/1

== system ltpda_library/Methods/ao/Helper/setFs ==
  In1 : Inport  OutDataType=sfix(16)  OutScaling=2^0
  setFs : M-S-Function  Tag=setFs  FunctionName=ltpdasim
  Out1 : Outport  OutDataType=sfix(16)  OutScaling=2^0
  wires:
  In1/1 -> setFs/1
  setFs/1 -> Out1/1

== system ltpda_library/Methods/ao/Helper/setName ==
  In1 : Inport  OutDataType=sfix(16)  OutScaling=2^0
  setName : M-S-Function  Tag=setName  FunctionName=ltpdasim
  Out1 : Outport  OutDataType=sfix(16)  OutScaling=2^0
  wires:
  In1/1 -> setName/1
  setName/1 -> Out1/1

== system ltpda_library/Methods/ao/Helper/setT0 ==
  In1 : Inport  OutDataType=sfix(16)  OutScaling=2^0
  setT0 : M-S-Function  Tag=setT0  FunctionName=ltpdasim
  Out1 : Outport  OutDataType=sfix(16)  OutScaling=2^0
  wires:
  In1/1 -> setT0/1
  setT0/1 -> Out1/1

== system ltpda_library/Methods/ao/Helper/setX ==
  In1 : Inport  OutDataType=sfix(16)  OutScaling=2^0
  setX : M-S-Function  Tag=setX  FunctionName=ltpdasim
  Out1 : Outport  OutDataType=sfix(16)  OutScaling=2^0
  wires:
  In1/1 -> setX/1
  setX/1 -> Out1/1

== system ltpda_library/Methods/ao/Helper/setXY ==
  In1 : Inport  OutDataType=sfix(16)  OutScaling=2^0
  setXY : M-S-Function  Tag=setXY  FunctionName=ltpdasim
  Out1 : Outport  OutDataType=sfix(16)  OutScaling=2^0
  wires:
  In1/1 -> setXY/1
  setXY/1 -> Out1/1

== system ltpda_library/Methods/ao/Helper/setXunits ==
  In1 : Inport  OutDataType=sfix(16)  OutScaling=2^0
  setXunits : M-S-Function  Tag=setXunits  FunctionName=ltpdasim
  Out1 : Outport  OutDataType=sfix(16)  OutScaling=2^0
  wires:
  In1/1 -> setXunits/1
  setXunits/1 -> Out1/1

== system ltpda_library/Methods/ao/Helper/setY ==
  In1 : Inport  OutDataType=sfix(16)  OutScaling=2^0
  setY : M-S-Function  Tag=setY  FunctionName=ltpdasim
  Out1 : Outport  OutDataType=sfix(16)  OutScaling=2^0
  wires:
  In1/1 -> setY/1
  setY/1 -> Out1/1

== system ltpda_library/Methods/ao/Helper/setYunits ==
  In1 : Inport  OutDataType=sfix(16)  OutScaling=2^0
  setYunits : M-S-Function  Tag=setYunits  FunctionName=ltpdasim
  Out1 : Outport  OutDataType=sfix(16)  OutScaling=2^0
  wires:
  In1/1 -> setYunits/1
  setYunits/1 -> Out1/1

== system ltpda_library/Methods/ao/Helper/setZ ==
  In1 : Inport  OutDataType=sfix(16)  OutScaling=2^0
  setZ : M-S-Function  Tag=setZ  FunctionName=ltpdasim
  Out1 : Outport  OutDataType=sfix(16)  OutScaling=2^0
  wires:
  In1/1 -> setZ/1
  setZ/1 -> Out1/1

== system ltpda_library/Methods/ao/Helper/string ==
  In1 : Inport  OutDataType=sfix(16)  OutScaling=2^0
  string : M-S-Function  Tag=string  FunctionName=ltpdasim
  Out1 : Outport  OutDataType=sfix(16)  OutScaling=2^0
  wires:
  In1/1 -> string/1
  string/1 -> Out1/1
